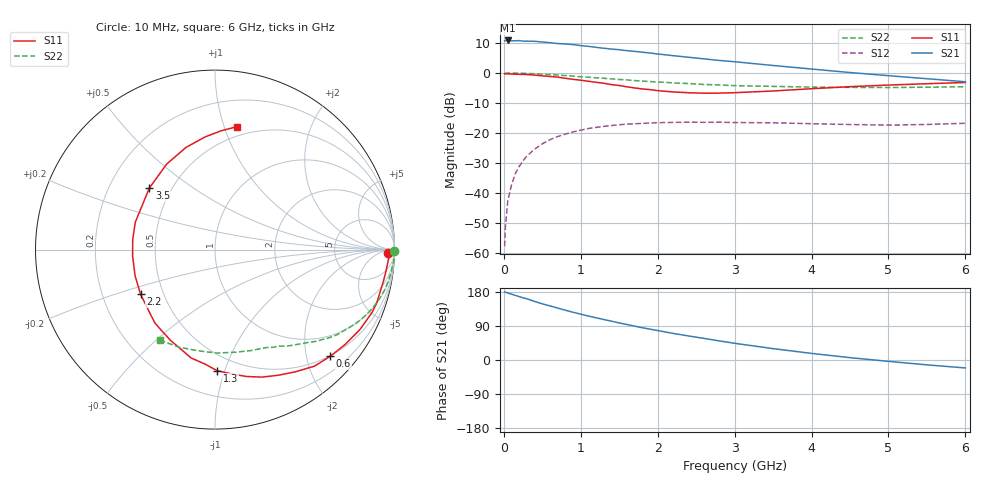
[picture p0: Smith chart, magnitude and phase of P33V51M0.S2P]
! SIEMENS Small Signal Semiconductors
! BFP181
! Si NPN RF Bipolar Junction Transistor in SOT143
! VCE = 3.5 V  IC = 1 mA
! Common Emitter S-Parameters:  March  1996
# GHz  S  MA  R  50
!  f  S11  S21  S12  S22
! GHz  MAG  ANG  MAG  ANG  MAG  ANG  MAG  ANG
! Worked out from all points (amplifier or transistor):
!   36 points, 10 MHz to 6 GHz, reference 50 ohm
!   highest |S21| = 10.8 dB at 50 MHz (marker M1)
!   |S21| within 3 dB of that: start of sweep to 1.46 GHz
!   unconditionally stable (mu >= 1): 3.138 GHz to end of sweep
!   at 250 MHz: K = 0.09, MSG = 19.9 dB, |S12| = -29.2 dB
!   at 1.4 GHz: K = 0.49, MSG = 12.7 dB, |S12| = -17.5 dB
!   at 6 GHz: K = 1.29, MAG = 3.7 dB, |S12| = -16.8 dB
!   lowest NFmin = 1.30 dB at 450 MHz
!   S11 on the Smith chart (normalised r, x): 10 MHz: 45, -22; 600 MHz: 0.49, -2.47; 1.3 GHz: 0.38, -0.94; 2.2 GHz: 0.37, -0.24; 3.5 GHz: 0.38, +0.35; 6 GHz: 0.42, +1.10
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0.01  0.9645 -1.0  3.445 179.6  0.0013 86.0  0.9985 -0.3
0.02  0.9732 -1.6  3.466 179.2  0.0027 93.6  0.9926 -0.6
0.05  0.9673 -3.5  3.485 176.8  0.0072 89.4  0.9962 -1.8
0.1  0.9602 -7.2  3.435 173.8  0.0137 83.7  0.9993 -3.4
0.15  0.9544 -10.9  3.444 170.5  0.0212 81.6  0.9931 -5.1
0.2  0.9496 -14.7  3.464 167.2  0.0277 80.2  0.9905 -6.8
0.25  0.9488 -18.3  3.392 164.0  0.0345 78.2  0.9855 -8.5
0.4  0.9222 -28.9  3.373 154.5  0.0538 71.1  0.9715 -13.4
0.6  0.875 -42.8  3.204 142.7  0.0773 61.9  0.9416 -19.4
0.9  0.784 -63.2  2.971 125.9  0.1043 49.8  0.8866 -27.6
1.1  0.7278 -76.2  2.78 115.9  0.1189 42.9  0.8489 -32.1
1.3  0.6745 -89.0  2.585 106.8  0.1291 36.6  0.8153 -36.4
1.5  0.6186 -102.4  2.444 97.8  0.1372 31.3  0.7796 -40.0
1.8  0.5422 -122.8  2.223 85.1  0.1448 24.6  0.7335 -44.8
2.2  0.4834 -149.1  1.945 70.2  0.1502 16.8  0.6857 -51.0
2.8  0.4619 172.9  1.618 50.4  0.1513 8.3  0.6322 -59.5
3  0.4697 161.0  1.54 44.1  0.1494 6.0  0.6158 -62.4
3.5  0.5012 136.9  1.334 30.0  0.1478 2.0  0.5979 -70.1
4  0.5469 119.6  1.164 17.4  0.1428 -0.8  0.5826 -79.1
4.5  0.5917 105.9  1.018 6.2  0.1384 -2.3  0.5763 -89.3
5.5  0.6627 87.1  0.803 -12.8  0.1387 0.9  0.5793 -110.3
6  0.6948 80.0  0.714 -21.0  0.1453 1.6  0.5906 -121.3
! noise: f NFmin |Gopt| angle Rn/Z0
0.45  1.3  0.7  18  0.5
0.9  1.4  0.6  39  0.52
1.8  1.85  0.4  81  0.47
